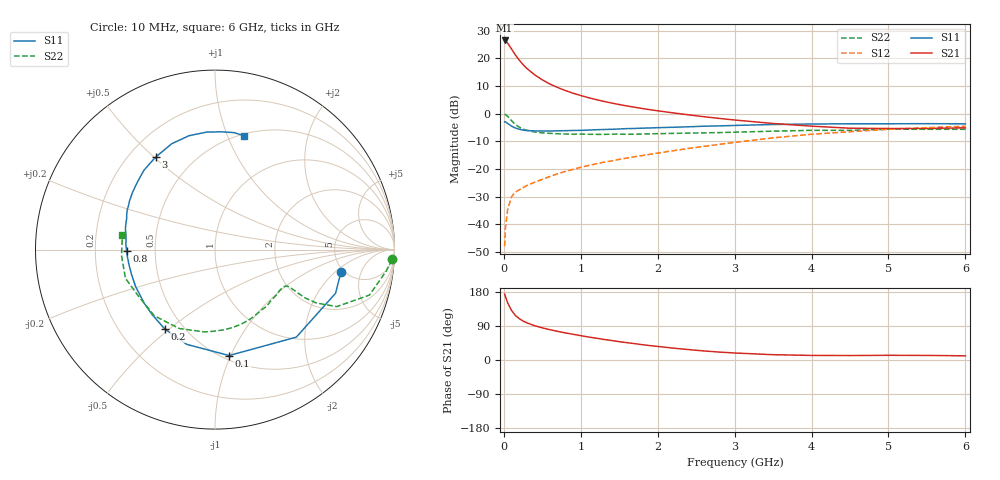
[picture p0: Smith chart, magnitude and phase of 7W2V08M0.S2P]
! Infineon Technologies  Discrete & RF Semiconductors
! BFS17W
! Si NPN RF Bipolar Junction Transistor in SOT323
! VCE = 2 V  IC = 8 mA
! Common Emitter S-Parameters:  August  1999
# GHz  S  MA  R  50
!  f  S11  S21  S12  S22
! GHz  MAG  ANG  MAG  ANG  MAG  ANG  MAG  ANG
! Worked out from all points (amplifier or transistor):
!   36 points, 10 MHz to 6 GHz, reference 50 ohm
!   highest |S21| = 26.5 dB at 10 MHz (marker M1)
!   |S21| within 3 dB of that: start of sweep to 97.89 MHz
!   unconditionally stable (mu >= 1): 414.8 MHz to 3.045 GHz; 4.041 GHz to end of sweep
!   at 250 MHz: K = 0.75, MSG = 22.3 dB, |S12| = -26.8 dB
!   at 1.4 GHz: K = 1.25, MAG = 7.4 dB, |S12| = -17.1 dB
!   at 6 GHz: K = 1.09, MAG = -2.1 dB, |S12| = -4.5 dB
!   S11 on the Smith chart (normalised r, x): 10 MHz: 4.75, -2.37; 100 MHz: 0.54, -0.99; 200 MHz: 0.40, -0.48; 800 MHz: 0.34, -0.00; 3 GHz: 0.31, +0.51; 6 GHz: 0.51, +1.15
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0.01  0.7132 -9.9  21.17 174.2  0.004 85.0  0.9872 -3.2
0.02  0.7144 -19.9  20.91 167.6  0.0083 87.1  0.9609 -7.2
0.05  0.6657 -47.1  18.97 150.7  0.0187 69.2  0.8972 -16.4
0.1  0.5954 -82.4  14.83 130.7  0.0312 57.4  0.749 -25.1
0.15  0.551 -106.6  11.57 117.6  0.0382 51.1  0.6376 -27.8
0.2  0.5231 -122.4  9.333 109.1  0.0418 51.0  0.5708 -28.2
0.25  0.5039 -134.0  7.731 102.9  0.0458 49.8  0.5257 -27.7
0.3  0.4952 -142.5  6.578 98.1  0.0502 51.0  0.5003 -27.3
0.4  0.488 -155.0  5.059 90.5  0.0574 53.2  0.4658 -26.7
0.5  0.4852 -163.4  4.098 84.8  0.0649 56.0  0.4502 -26.8
0.6  0.4864 -169.7  3.436 79.9  0.0732 57.4  0.4404 -27.6
0.7  0.4893 -174.8  2.977 75.6  0.0818 59.4  0.4334 -29.1
0.8  0.4929 -179.4  2.625 71.5  0.0902 60.3  0.4288 -31.0
1.1  0.5054 169.6  1.95 60.7  0.1153 62.1  0.4243 -37.7
1.3  0.5175 163.5  1.671 54.3  0.1324 63.0  0.422 -43.2
1.6  0.5371 155.5  1.381 45.7  0.1576 63.5  0.4241 -51.7
2.2  0.568 141.1  1.035 31.4  0.2136 63.8  0.4404 -70.7
3  0.6125 122.6  0.769 18.5  0.3027 60.5  0.4622 -97.2
3.5  0.6373 112.2  0.665 14.0  0.3654 56.1  0.4828 -114.4
4.5  0.6566 93.9  0.546 11.8  0.4714 43.8  0.4989 -148.4
5.5  0.6603 80.9  0.54 12.1  0.5588 31.8  0.5221 -176.5
6  0.6554 75.9  0.555 11.0  0.5929 26.0  0.5218 171.2
